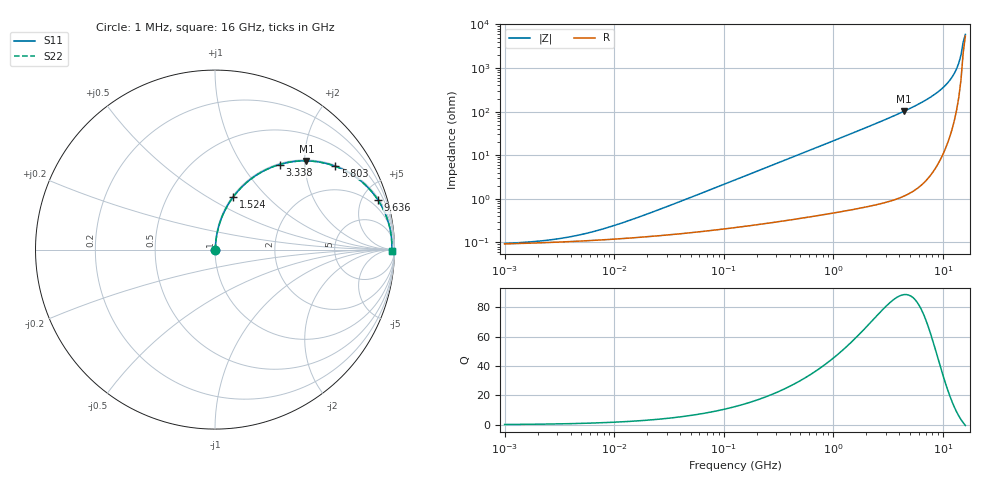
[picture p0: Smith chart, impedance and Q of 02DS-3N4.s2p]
# MHz S MA R 50
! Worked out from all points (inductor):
!   211 points, 1 MHz to 16 GHz, reference 50 ohm
!   read as one part in series: L = 3.4 nH near 19.11 MHz
!   highest Q = 88.3 at 4.401 GHz (marker M1), where L = 3.69 nH
!   self-resonance near 15.28 GHz
!   S11 on the Smith chart (normalised r, x): 1 MHz: 1.00, +0.00; 1.524 GHz: 1.01, +0.66; 3.338 GHz: 1.02, +1.49; 5.803 GHz: 1.03, +2.87; 9.636 GHz: 1.17, +6.54; 16 GHz: open
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1  0.0009465 13.0  0.9991 -0.0  0.9991 -0.0  0.0009465 13.0
2.51416  0.00113 28.3  0.999 -0.0  0.999 -0.0  0.00113 28.3
5.25662  0.001558 46.0  0.9989 -0.1  0.9989 -0.1  0.001558 46.0
10.4954  0.002539 61.7  0.9988 -0.1  0.9988 -0.1  0.002539 61.7
26.3872  0.005808 75.4  0.9986 -0.3  0.9986 -0.3  0.005808 75.4
132.458  0.02831 83.9  0.9974 -1.6  0.9974 -1.6  0.02831 83.9
333.021  0.07085 83.5  0.9945 -4.1  0.9945 -4.1  0.07085 83.5
664.915  0.1404 80.3  0.9862 -8.1  0.9862 -8.1  0.1404 80.3
1524.47  0.3107 70.9  0.9451 -18.1  0.9451 -18.1  0.3107 70.9
2204.33  0.4305 63.7  0.8964 -25.5  0.8964 -25.5  0.4305 63.7
3187.38  0.5755 54.2  0.8108 -35.1  0.8108 -35.1  0.5755 54.2
3337.74  0.5947 52.8  0.7968 -36.5  0.7968 -36.5  0.5947 52.8
4401.2  0.7098 44.1  0.6964 -45.2  0.6964 -45.2  0.7098 44.1
5803.48  0.8155 34.7  0.5691 -54.6  0.5691 -54.6  0.8155 34.7
7652.55  0.9001 24.9  0.4216 -64.1  0.4216 -64.1  0.9001 24.9
9636.16  0.9493 16.9  0.29 -71.6  0.29 -71.6  0.9493 16.9
11587.3  0.9738 10.5  0.1825 -76.5  0.1825 -76.5  0.9738 10.5
13305.8  0.9834 5.8  0.1019 -77.7  0.1019 -77.7  0.9834 5.8
13933.5  0.9849 4.3  0.0753 -76.3  0.0753 -76.3  0.9849 4.3
14590.9  0.9856 2.7  0.04917 -71.6  0.04917 -71.6  0.9856 2.7
15279.2  0.9855 1.2  0.02497 -53.9  0.02497 -53.9  0.9855 1.2
16000  0.9846 -0.4  0.01668 22.0  0.01668 22.0  0.9846 -0.4
